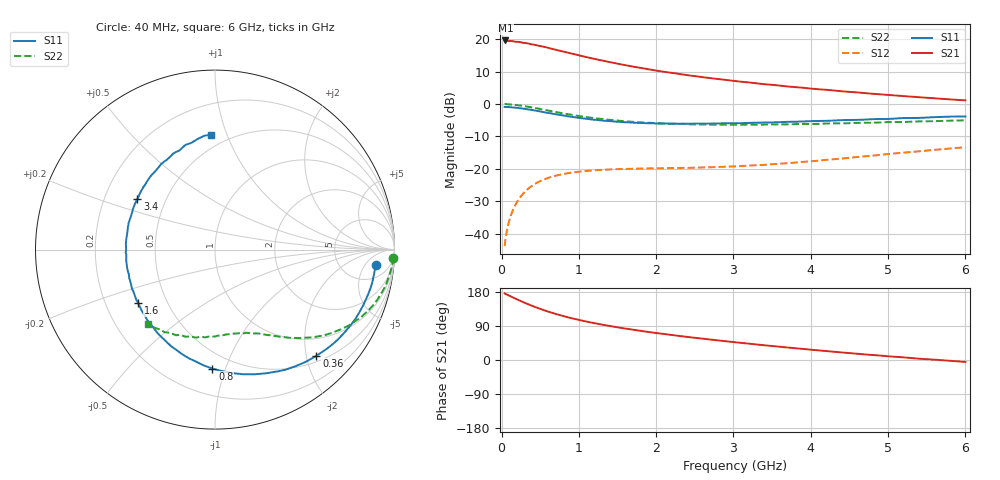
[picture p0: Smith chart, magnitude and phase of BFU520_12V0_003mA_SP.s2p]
! Filename:  P:\Prog\Test\Noise\ATS_data\Testdata_Net\03 Spar\BFU520_APG2013_37_A05_12p0V_003mA_SP_CM01_D.s2p
! Date/Time: Fri 26/Apr/2013 13:00:11
! BFU520_APG2013_37_A05_12p0V_1to20mA_SP_CM01_Bias3_R.s2p
! MDIF S-parameter v. bias file
! BFU520_APG2013_37_A05_12p0V_1to20mA_SP_CM01
! Date/time Tue Apr 23 18:22:57 2013
! VAR V_out= 12.0010
! VAR I_out= 3.0100
! VAR V_in= 0.8064
! VAR I_in= 0.0276
! Device data file deembeded for feedlines and parallel
! Original file: \03 Spar\BFU520_APG2013_37_A05_12p0V_003mA_SP_CM01_R.s2p
! Feed-files: PR047V01_250413_Feed1.s2p, PR047V01_250413_Feed2.s2p
! Parallel-file: PR047V01_250413_Par.s2p
# MHz S MA R 50
!  Freq-MHz  S11-mag  S11-arg  S21-mag  S21-arg  S12-mag  S12-arg  S22-mag  S22-arg
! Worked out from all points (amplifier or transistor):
!   98 points, 40 MHz to 6 GHz, reference 50 ohm
!   highest |S21| = 19.6 dB at 50 MHz (marker M1)
!   |S21| within 3 dB of that: start of sweep to 725.5 MHz
!   unconditionally stable (mu >= 1): 2.755 GHz to 4.697 GHz
!   at 300 MHz: K = 0.14, MSG = 23.0 dB, |S12| = -27.2 dB
!   at 1.6 GHz: K = 0.64, MSG = 16.0 dB, |S12| = -20.0 dB
!   at 6 GHz: K = 0.83, MSG = 7.2 dB, |S12| = -13.3 dB
!   S11 on the Smith chart (normalised r, x): 40 MHz: 11, -9; 360 MHz: 0.61, -2.20; 800 MHz: 0.38, -0.90; 1.6 GHz: 0.34, -0.28; 3.4 GHz: 0.34, +0.26; 6 GHz: 0.41, +0.88
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40  0.9004 -5.4  9.506 175.8  0.006407 84.2  0.9933 -2.6
50  0.8986 -6.7  9.527 174.2  0.008025 84.1  0.9955 -3.5
70  0.8963 -9.2  9.411 172.9  0.01114 83.2  0.9896 -5.1
90  0.8946 -11.9  9.319 170.6  0.01427 81.9  0.987 -6.5
120  0.8894 -16.0  9.366 167.7  0.01894 79.9  0.9813 -8.7
240  0.859 -31.6  8.991 156.3  0.03626 71.2  0.9473 -17.1
360  0.8181 -46.3  8.472 145.9  0.05094 63.5  0.8995 -24.5
440  0.7894 -55.5  8.099 139.4  0.05914 58.9  0.8628 -28.8
550  0.7453 -67.7  7.592 131.2  0.06833 53.1  0.8121 -34.1
700  0.6937 -82.4  6.872 121.6  0.07807 46.9  0.7511 -40.0
800  0.6631 -91.3  6.418 115.9  0.08304 43.6  0.7137 -43.4
900  0.633 -99.7  6.007 110.6  0.08712 40.7  0.6821 -46.3
1050  0.5988 -111.2  5.446 103.5  0.09137 37.1  0.6384 -50.3
1300  0.5552 -127.8  4.677 93.4  0.0963 32.9  0.5848 -55.4
1600  0.5214 -145.2  3.964 83.0  0.09944 29.8  0.5402 -60.8
2050  0.5005 -166.0  3.198 70.0  0.1016 28.4  0.5014 -67.8
2500  0.4978 176.5  2.686 58.7  0.1041 29.3  0.4839 -74.6
3100  0.5055 156.2  2.202 45.2  0.1102 33.0  0.478 -83.8
3400  0.5162 146.9  2.015 38.9  0.1151 34.8  0.4806 -88.7
4100  0.5465 129.2  1.684 25.4  0.1335 38.8  0.4933 -99.8
5200  0.606 105.8  1.321 7.0  0.1773 39.5  0.5262 -118.2
6000  0.6404 92.0  1.135 -5.1  0.2153 36.0  0.5592 -131.8
